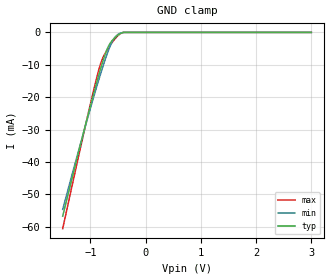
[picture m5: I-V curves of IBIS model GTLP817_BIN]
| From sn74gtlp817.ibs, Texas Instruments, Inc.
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[Model]   GTLP817_BIN
Model_type  Input
Vinl=0.95
Vinh=1.05
| variable   typ   min   max
C_comp   2.95pF   2.44pF   3.35pF
[Temperature Range]   40   100   -40
| Ambient temperature   25   85   -40
[Voltage range]   1.5   1.5   1.5
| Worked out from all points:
|   GND clamp passes 1 mA (typ) near -0.51 V on its own axis
[GND Clamp]
| GTLP817_BIN
|   Voltage   I(typ)   I(min)   I(max)
-1.5V     -56.78mA   -54.68mA   -60.62mA
-1.065V   -27.06mA   -27.47mA   -27.04mA
-920mV    -17.67mA   -18.83mA   -16.45mA
-835mV    -12.45mA   -13.97mA   -10.86mA
-770mV    -8.748mA   -10.42mA   -7.731mA
-715mV    -6.002mA   -7.591mA   -5.977mA
-670mV    -4.221mA   -5.468mA   -4.738mA
-620mV    -2.847mA   -3.424mA   -3.472mA
-575mV    -1.965mA   -2.005mA   -2.439mA
-475mV    -541.8uA   -380uA     -635.4uA
-390mV    -8.736uA   -22.02uA   -7.093uA
3V        158.5pA    570.4pA    1.278nA
